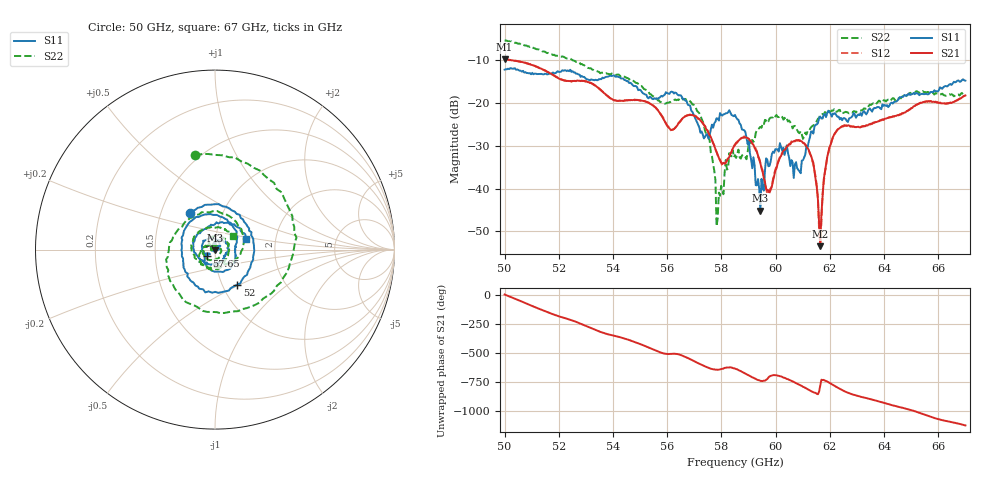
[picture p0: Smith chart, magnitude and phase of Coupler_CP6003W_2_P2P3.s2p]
!Agilent Technologies,E8361A,US42410132,A.06.03.05
!Agilent E8361A: A.06.03.05
!Date: Friday, July 11, 2008 16:51:09
!Correction: S11(Full 2 Port(1,2)) S21(Full 2 Port(1,2)) S12(Full 2 Port(1,2)) S22(Full 2 Port(1,2))
!S2P File: Measurements: S11, S21, S12, S22:
# Hz S  MA  R 50
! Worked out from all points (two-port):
!   401 points, 50 GHz to 67 GHz, reference 50 ohm
!   highest |S21| = -9.74 dB at 50 GHz (marker M1); lowest = -53.5 dB at 61.65 GHz (marker M2)
!   |S21| within 3 dB of the highest: start of sweep to 51.58 GHz
!   lowest |S11| = -45.1 dB at 59.44 GHz (marker M3), VSWR 1.01, Z = 50.2 - j0.499 ohm
!   |S11| at or under -10 dB: start of sweep to end of sweep
!   |S22| runs from -48.8 to -5.4 dB; largest |S21 - S12| = 0.0062
!   S11 on the Smith chart (normalised r, x): 50 GHz: 0.70, +0.30; 52 GHz: 1.18, -0.48; 57.65 GHz: 0.91, -0.06; 67 GHz: 1.41, +0.17
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5e10  0.2455 124.9  0.3259 2.4  0.3293 2.6  0.5383 101.9
5.0935e10  0.2239 31.8  0.2837 -88.1  0.2852 -88.1  0.4508 12.2
5.19975e10  0.2312 -57.3  0.1932 175.4  0.1955 175.7  0.3551 -85.4
5.28475e10  0.2069 -142.9  0.183 107.7  0.1816 107.8  0.2861 -160.0
5.41225e10  0.2038 111.7  0.1064 2.4  0.1062 2.9  0.2141 93.4
5.5695e10  0.1148 -9.7  0.07904 -131.8  0.07915 -131.8  0.1072 -47.0
5.61625e10  0.1358 -51.9  0.04836 -148.7  0.04848 -148.9  0.1044 -71.0
5.69275e10  0.07884 -136.1  0.07278 155.5  0.072 155.9  0.09607 -150.2
5.765e10  0.05594 -142.6  0.03689 80.6  0.0368 82.5  0.0239 121.0
5.7905e10  0.06236 -169.5  0.02287 75.0  0.02324 76.8  0.008973 132.5
5.85e10  0.07258 114.9  0.03239 84.1  0.03274 85.0  0.0246 132.9
5.89675e10  0.03307 44.9  0.03896 30.1  0.03811 30.7  0.02685 17.5
5.9435e10  0.005548 -63.6  0.01996 -21.3  0.01995 -22.6  0.05266 -72.7
5.97325e10  0.01823 158.8  0.009557 7.0  0.008576 1.2  0.06123 -107.5
6.05825e10  0.02153 66.4  0.03483 -21.2  0.03561 -22.4  0.05683 164.3
6.09225e10  0.01512 106.4  0.03604 -61.6  0.03643 -61.3  0.04686 147.8
6.13475e10  0.04667 92.6  0.02189 -115.1  0.02138 -116.1  0.05378 132.0
6.1645e10  0.06951 57.0  0.002125 -62.5  0.002237 -65.0  0.07288 105.7
6.19e10  0.07548 23.4  0.02312 -26.8  0.0229 -27.1  0.0764 77.8
6.224e10  0.0718 -9.6  0.04659 -74.3  0.04677 -74.5  0.07933 34.7
6.4195e10  0.09323 -140.8  0.06816 135.9  0.06758 135.6  0.11 -124.3
6.7e10  0.1826 18.9  0.1225 -45.9  0.1212 -45.8  0.1242 37.0
